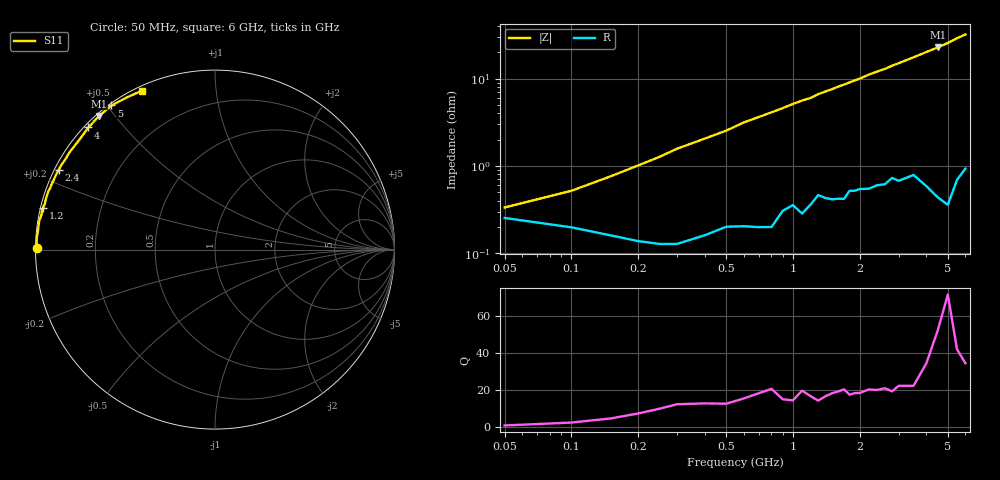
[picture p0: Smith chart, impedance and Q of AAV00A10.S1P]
! Infineon Technologies  Discrete & RF Semiconductors
! BBY66-02W
! Si Tuning Diode in SCD-80
! VR =
! S-Parameters:  June  2000
# GHz  S  MA  R  50
!  f  S11
! GHz  MAG  ANG
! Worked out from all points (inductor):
!   34 points, 50 MHz to 6 GHz, reference 50 ohm
!   read as one part to ground: L = 799 pH near 150 MHz
!   highest Q = 52 at 4.5 GHz (marker M1), where L = 806 pH
!   S11 on the Smith chart (normalised r, x): 50 MHz: 0.01, +0.00; 1.2 GHz: 0.01, +0.12; 2.4 GHz: 0.01, +0.24; 4 GHz: 0.01, +0.40; 5 GHz: 0.01, +0.51; 6 GHz: 0.02, +0.64
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0.05  0.9899 179.5
0.15  0.9936 178.3
0.25  0.9949 177.1
0.3  0.9949 176.4
0.5  0.992 174.2
0.6  0.9919 172.8
0.8  0.9921 170.6
1  0.986 168.3
1.1  0.9888 167.2
1.2  0.9859 166.3
1.3  0.9819 164.9
1.5  0.9839 162.8
1.6  0.9837 161.6
1.7  0.9838 160.6
1.8  0.9801 159.5
1.9  0.9801 158.4
2  0.9793 157.4
2.2  0.9793 154.9
2.4  0.9775 152.9
2.6  0.9771 151.0
2.8  0.9733 148.6
3  0.9755 146.5
3.5  0.9723 141.3
4  0.98 136.0
4.5  0.9856 131.0
5  0.9887 125.7
5.5  0.9795 119.7
6  0.9739 114.6
